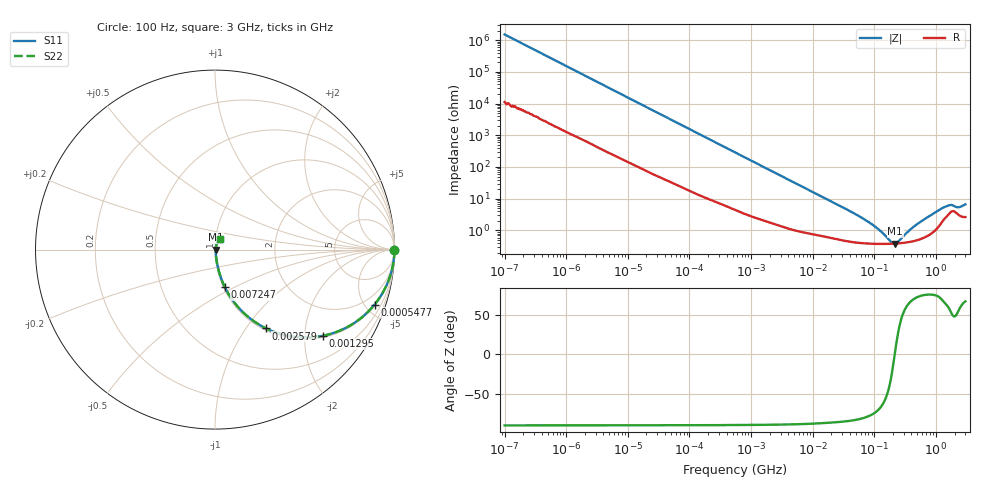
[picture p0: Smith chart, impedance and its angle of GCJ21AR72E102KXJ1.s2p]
!Murata Part Number: GCJ21AR72E102KXJ1
!These Parameters are Measured in Series Mode Connection
!Data Generated on Mar 13, 2026
!  o--ll--o
!Port1  Port2
!  o------o
!Operation Temp=25[degC], DC Bias Voltage=0[V]
!Freq. Start=100[Hz] Stop=3[GHz] 401[Steps]
# Hz S RI R 50
!Freq.(Hz) S11(Real) S11(Imag) S21(Real) S21(Imag) S12(Real) S12(Imag) S22(Real) S22(Imag)
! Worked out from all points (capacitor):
!   401 points, 100 Hz to 3 GHz, reference 50 ohm
!   read as one part in series: C = 1.06 nF near 109 Hz
!   lowest |Z| = 387 mohm at 217.2 MHz (marker M1)
!   series resonance near 214.2 MHz, so ESL is about 520 pH
!   S11 on the Smith chart (normalised r, x): 100 Hz: open; 547.7 kHz: 1.09, -5.78; 1.295 MHz: 1.05, -2.46; 2.579 MHz: 1.03, -1.25; 7.247 MHz: 1.02, -0.45; 3 GHz: 1.05, +0.12
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100  1 -6.66e-05  5e-07 6.66e-05  5e-07 6.66e-05  1 -6.66e-05
161  1 -0.000107  8e-07 0.000107  8e-07 0.000107  1 -0.000107
1788  1 -0.00117  1.16e-05 0.00117  1.16e-05 0.00117  1 -0.00117
31977  0.9994 -0.0206  0.000632 0.0206  0.000632 0.0206  0.9994 -0.0206
164120  0.9879 -0.1033  0.0121 0.1033  0.0121 0.1033  0.9879 -0.1033
547723  0.8895 -0.306  0.1105 0.306  0.1105 0.306  0.8895 -0.306
842342  0.7768 -0.4081  0.2232 0.4081  0.2232 0.4081  0.7768 -0.4081
1295438  0.6008 -0.4803  0.3992 0.4803  0.3992 0.4803  0.6008 -0.4803
2579298  0.2845 -0.4392  0.7155 0.4392  0.7155 0.4392  0.2845 -0.4392
4141163  0.1392 -0.3321  0.8608 0.3321  0.8608 0.3321  0.1392 -0.3321
7246509  0.0552 -0.2101  0.9448 0.2101  0.9448 0.2101  0.0552 -0.2101
9794414  0.034 -0.1597  0.966 0.1597  0.966 0.1597  0.034 -0.1597
7.093284e7  0.00434 -0.0211  0.9957 0.0211  0.9957 0.0211  0.00434 -0.0211
1.138854e8  0.00387 -0.0106  0.9961 0.0106  0.9961 0.0106  0.00387 -0.0106
1.751444e8  0.00379 -0.00319  0.9962 0.00319  0.9962 0.00319  0.00379 -0.00319
2.172002e8  0.00385 0.00022  0.9962 -0.00022  0.9962 -0.00022  0.00385 0.00022
2.471375e8  0.00392 0.00226  0.9961 -0.00226  0.9961 -0.00226  0.00392 0.00226
4.713361e8  0.00497 0.0138  0.995 -0.0138  0.995 -0.0138  0.00497 0.0138
1.214989e9  0.0187 0.0443  0.9813 -0.0443  0.9813 -0.0443  0.0187 0.0443
1.642185e9  0.0353 0.0491  0.9647 -0.0491  0.9647 -0.0491  0.0353 0.0491
2.317205e9  0.0319 0.0413  0.9681 -0.0413  0.9681 -0.0413  0.0319 0.0413
3e9  0.0292 0.0577  0.9708 -0.0577  0.9708 -0.0577  0.0292 0.0577
